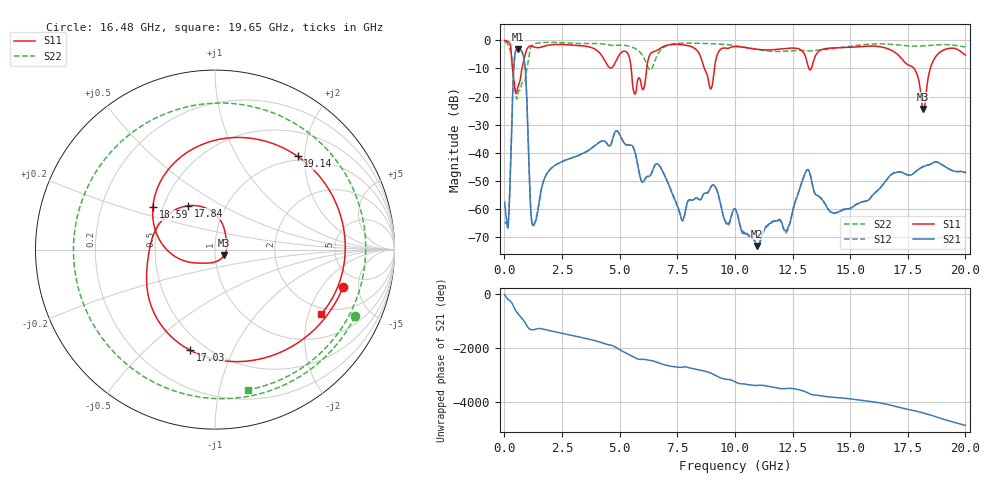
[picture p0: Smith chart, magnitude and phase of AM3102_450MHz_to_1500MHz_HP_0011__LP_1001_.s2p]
!Agilent Technologies,E8364B,MY43040894,A.07.50.67
!Agilent E8364B: A.07.50.67
!Date: Thursday, January 11, 2018 05:32:27
!Correction: S11(Full 2 Port(1,2))
!S21(Full 2 Port(1,2))
!S12(Full 2 Port(1,2))
!S22(Full 2 Port(1,2))
!S2P File: Measurements: S11, S21, S12, S22:
# Hz S  dB  R 50
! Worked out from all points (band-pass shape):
!   1601 points, 10 MHz to 20 GHz, reference 50 ohm
!   highest |S21| = -3.03 dB at 597.2 MHz (marker M1); lowest = -73.1 dB at 10.95 GHz (marker M2)
!   |S21| within 3 dB of the highest: 443.5 MHz to 838 MHz (394.5 MHz wide, 61.6 % of centre)
!   lowest |S11| = -24.4 dB at 18.18 GHz (marker M3), VSWR 1.13, Z = 55.3 - j3.55 ohm
!   |S11| at or under -10 dB: 5.501 GHz to 6.175 GHz (673.5 MHz wide, 11.5 % of centre); 8.68 GHz to 9.111 GHz (431.3 MHz wide, 4.85 % of centre); 17.77 GHz to 18.48 GHz (708.9 MHz wide, 3.91 % of centre)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
!   |S22| runs from -20.9 to -0.4 dB; largest |S21 - S12| = 0.0043
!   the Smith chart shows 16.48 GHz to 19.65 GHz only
!   S11 on the Smith chart (normalised r, x): 16.48 GHz: 3.57, -3.32; 17.03 GHz: 0.41, -0.69; 17.84 GHz: 0.67, +0.35; 18.59 GHz: 0.44, +0.25; 19.14 GHz: 0.92, +1.85; 19.65 GHz: 1.77, -2.44
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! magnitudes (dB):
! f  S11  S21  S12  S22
! 10 MHz  0.0  -57.5  -64.5  -0.4
! 172.4 MHz  -0.6  -65.1  -63.8  -1.9
! 422.3 MHz  -15.2  -8.0  -8.0  -14.1
! 597.2 MHz  -16.3  -3.0  -3.0  -18.5
! 884.6 MHz  -5.7  -8.3  -8.3  -14.6
! 1.259 GHz  -2.3  -65.7  -65.6  -1.5
! 3.346 GHz  -1.9  -40.4  -40.4  -1.1
! 5.657 GHz  -19.1  -39.5  -39.5  -2.8
! 6.682 GHz  -3.2  -44.1  -44.1  -4.6
! 7.706 GHz  -1.6  -63.8  -64.0  -1.0
! 10.01 GHz  -2.2  -60.0  -59.9  -1.9
! 10.95 GHz  -3.2  -73.1  -72.9  -3.2
! 13.34 GHz  -9.4  -50.5  -50.5  -3.7
! 16.48 GHz  -2.6  -50.7  -50.7  -1.3
! 16.68 GHz  -3.1  -48.5  -48.6  -1.4
! 17.03 GHz  -4.8  -46.9  -46.8  -1.6
! 17.84 GHz  -10.9  -46.7  -46.6  -2.1
! 18.18 GHz  -24.4  -44.8  -44.8  -2.0
! 18.59 GHz  -7.6  -43.5  -43.5  -1.7
! 19.14 GHz  -3.2  -45.0  -45.0  -1.5
! 19.65 GHz  -3.2  -46.6  -46.6  -1.9
! 20 GHz  -5.2  -47.0  -47.1  -2.3
